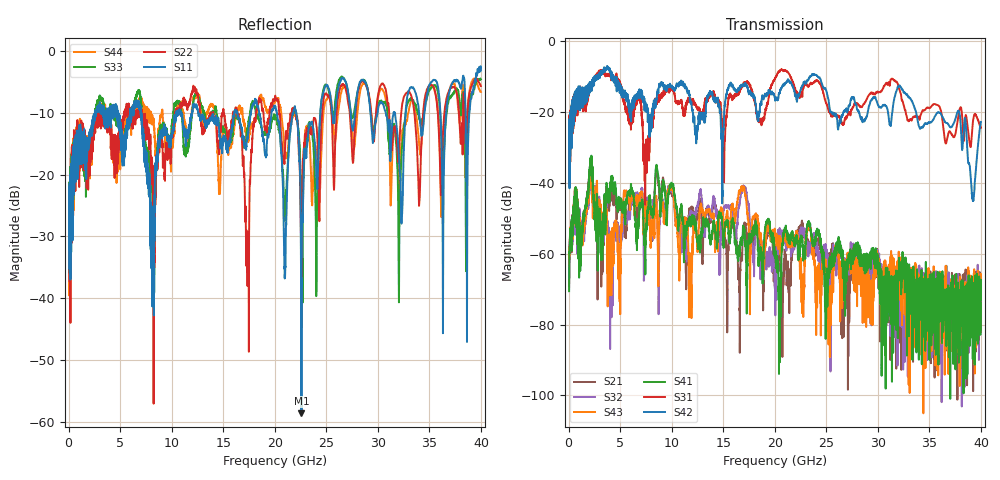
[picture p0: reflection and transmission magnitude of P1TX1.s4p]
!Agilent Technologies,N5245A,MY49151084,A.09.20.08
!Agilent N5245A: A.09.20.08
!Date: Thursday, March 01, 2012 14:41:56
!Correction: S11(Full 4 Port(1,2,3,4))
!S12(Full 4 Port(1,2,3,4))
!S13(Full 4 Port(1,2,3,4))
!S14(Full 4 Port(1,2,3,4))
!S21(Full 4 Port(1,2,3,4))
!S22(Full 4 Port(1,2,3,4))
!S23(Full 4 Port(1,2,3,4))
!S24(Full 4 Port(1,2,3,4))
!S31(Full 4 Port(1,2,3,4))
!S32(Full 4 Port(1,2,3,4))
!S33(Full 4 Port(1,2,3,4))
!S34(Full 4 Port(1,2,3,4))
!S41(Full 4 Port(1,2,3,4))
!S42(Full 4 Port(1,2,3,4))
!S43(Full 4 Port(1,2,3,4))
!S44(Full 4 Port(1,2,3,4))
!S4P File: Measurements: <S11,S12,S13,S14>,
!<S21,S22,S23,S24>,
!<S31,S32,S33,S34>,
!<S41,S42,S43,S44>:
# Hz S  dB  R 50
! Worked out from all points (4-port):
!   3996 points, 50 MHz to 40 GHz, reference 50 ohm
!   strongest paths, dB at 50 MHz, 10.04 GHz, 20.03 GHz, 30.02 GHz, 40 GHz:
!     S42: -26.6, -12.9, -16.6, -17.9, -22.8
!     S31: -23.6, -13.7, -10.6, -14.5, -24.4
!     S41: -70.6, -40.9, -61.2, -63.3, -73.0
!     S43: -60.5, -42.0, -54.5, -62.9, -67.1
!     S32: -60.7, -42.6, -65.4, -63.1, -69.7
!     S21: -69.2, -43.5, -62.6, -63.8, -77.0
!   lowest |S11| = -58.7 dB at 22.59 GHz (marker M1), VSWR 1.00, Z = 50 - j0.116 ohm
!   |S11| at or under -10 dB: start of sweep to 2.585 GHz; 7.041 GHz to 10.46 GHz (3.414 GHz wide, 39 % of centre); 12.58 GHz to 16.07 GHz (3.491 GHz wide, 24.4 % of centre)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
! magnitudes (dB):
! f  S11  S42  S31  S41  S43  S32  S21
! 50 MHz  -23.8  -26.6  -23.6  -70.6  -60.5  -60.7  -69.2
! 2.15 GHz  -13.3  -12.9  -13.5  -34.3  -38.3  -38.9  -35.2
! 4.12 GHz  -9.6  -8.7  -9.3  -40.1  -65.7  -74.9  -42.5
! 7.43 GHz  -16.6  -18.1  -46.2  -61.5  -47.9  -50.4  -57.6
! 16.88 GHz  -13.8  -12.5  -12.7  -55.6  -42.0  -41.7  -56.9
! 22.59 GHz  -58.7  -13.0  -14.9  -55.0  -66.2  -54.3  -52.1
! 40 GHz  -3.1  -22.8  -24.4  -73.0  -67.1  -69.7  -77.0
